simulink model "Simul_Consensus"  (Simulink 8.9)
settings: Solver=ode45  StartTime=0.0  StopTime=Tf  MaxStep=0.1  RelTol=1e-3  EnableMultiTasking=on
undefined symbols (not defined in the file or in its folder): K, Tc

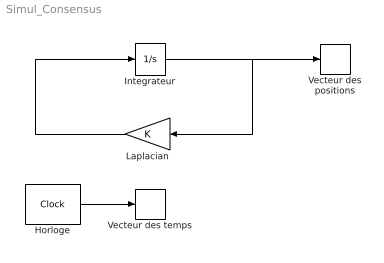
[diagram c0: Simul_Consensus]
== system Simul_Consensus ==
  Horloge : Clock
  Integrateur : Integrator  ZeroCross=off
  Laplacian : Gain  Gain=K  Multiplication=Matrix(K*u) (u vector)  SampleTime=Tc
  Vecteur des positions : ToWorkspace  VariableName=x  SampleTime=Tc
  Vecteur des temps : ToWorkspace  VariableName=T  SampleTime=Tc
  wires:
  Laplacian/1 -> Integrateur/1
  Integrateur/1 -> Vecteur des positions/1, Laplacian/1
  Horloge/1 -> Vecteur des temps/1
